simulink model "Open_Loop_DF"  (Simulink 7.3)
settings: Solver=ode3  StartTime=0.0  StopTime=500  FixedStep=0.002  RelTol=1e-3
undefined symbols (not defined in the file or in its folder): Acs, Av1, Bcs, Bv1, Ccs, Cv1, Dcs, Dv1

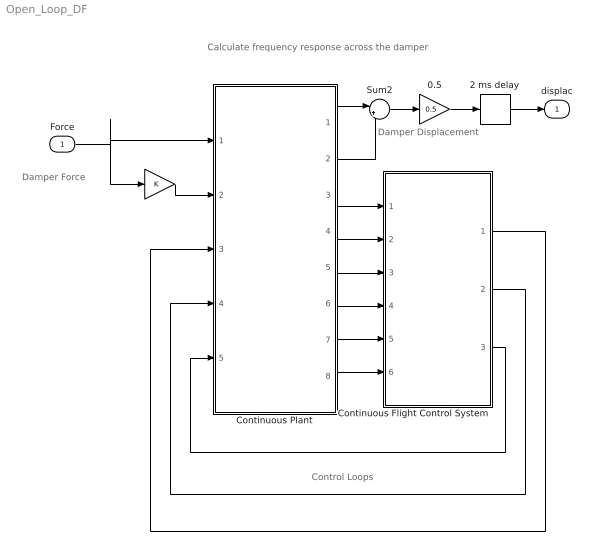
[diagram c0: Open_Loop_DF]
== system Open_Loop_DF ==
  note: Calculate frequency response across the damper
  note: Control Loops
  note: Damper Force
  note: Damper Displacement
  Force : Inport  OutDataType=sfix(16)  OutScaling=2^0
  "  " : Gain  ParameterDataType=sfix(16)  ParameterScaling=2^0  OutDataType=sfix(16)  OutScaling=2^0
  0.5 : Gain  Gain=0.5  ParameterDataType=sfix(16)  ParameterScaling=2^0  OutDataType=sfix(16)  OutScaling=2^0
  2 ms delay : TransportDelay  DelayTime=0.002  PadeOrder=2
  Continuous Flight Control System : Subsystem
  Continuous Plant : Subsystem
  Sum2 : Sum  Inputs=|++  OutDataType=sfix(16)  OutScaling=2^0
  displac : Outport  OutDataType=sfix(16)  OutScaling=2^0
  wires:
  Force/1 -> "  "/1, Continuous Plant/1(F-left)
  Sum2/1 -> 0.5/1
  0.5/1 -> 2 ms delay/1
  "  "/1 -> Continuous Plant/2(F-right)
  Continuous Plant/3(phi) -> Continuous Flight Control System/1(Phi)
  Continuous Plant/4(theta) -> Continuous Flight Control System/2(Theta)
  Continuous Plant/6(P) -> Continuous Flight Control System/4(P)
  Continuous Plant/7(Q) -> Continuous Flight Control System/5(Q)
  Continuous Plant/8(R) -> Continuous Flight Control System/6(R)
  Continuous Plant/5(psi) -> Continuous Flight Control System/3(Psi)
  Continuous Flight Control System/2(DQ-TVC) -> Continuous Plant/4(DQ)
  Continuous Flight Control System/3(DR-TVC) -> Continuous Plant/5(DR)
  Continuous Flight Control System/1(DP-TVC) -> Continuous Plant/3(DP)
  2 ms delay/1 -> displac/1
  Continuous Plant/1(dZ-Left) -> Sum2/1
  Continuous Plant/2(dZ-Rght) -> Sum2/2

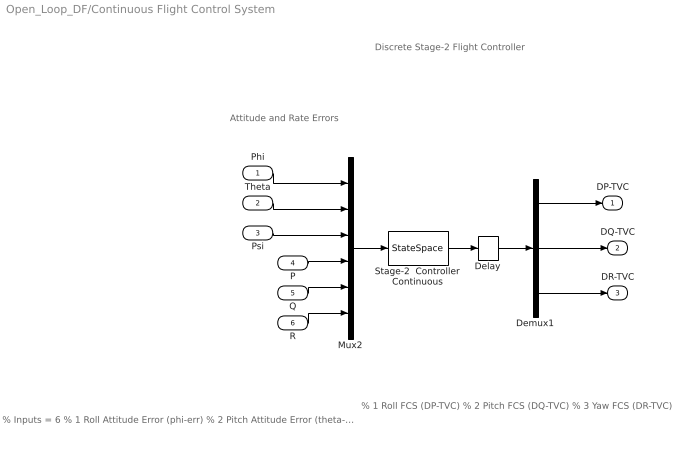
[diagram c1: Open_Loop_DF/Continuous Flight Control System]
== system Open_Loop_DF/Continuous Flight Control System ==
  note: % 1 Roll FCS (DP-TVC) % 2 Pitch FCS (DQ-TVC) % 3 Yaw FCS (DR-TVC)
  note: % Inputs = 6 % 1 Roll Attitude Error (phi-err) % 2 Pitch Attitude Error (theta-err) % 3 Yaw Attitude Error (psi-err) % 4 Roll Rate Error (p-err) % 5 Pitch Rate Error (q-err) % 6 Yaw Rate Error (r-err)
  note: Attitude and Rate Errors
  note: Discrete Stage-2 Flight Controller
  Phi : Inport  OutDataType=sfix(16)  OutScaling=2^0
  Theta : Inport  Port=2  OutDataType=sfix(16)  OutScaling=2^0
  Psi : Inport  Port=3  OutDataType=sfix(16)  OutScaling=2^0
  P : Inport  Port=4  OutDataType=sfix(16)  OutScaling=2^0
  Q : Inport  Port=5  OutDataType=sfix(16)  OutScaling=2^0
  R : Inport  Port=6  OutDataType=sfix(16)  OutScaling=2^0
  Delay : TransportDelay  DelayTime=0.04  PadeOrder=2
  Demux1 : Demux  Outputs=3
  Mux2 : Mux  Inputs=6
  Stage-2  Controller Continuous : StateSpace  A=Acs  B=Bcs  C=Ccs  D=Dcs
  DP-TVC : Outport  OutDataType=sfix(16)  OutScaling=2^0
  DQ-TVC : Outport  Port=2  OutDataType=sfix(16)  OutScaling=2^0
  DR-TVC : Outport  Port=3  OutDataType=sfix(16)  OutScaling=2^0
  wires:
  Demux1/3 -> DR-TVC/1
  Demux1/1 -> DP-TVC/1
  Demux1/2 -> DQ-TVC/1
  P/1 -> Mux2/4
  Stage-2  Controller Continuous/1 -> Delay/1
  Psi/1 -> Mux2/3
  Theta/1 -> Mux2/2
  Phi/1 -> Mux2/1
  R/1 -> Mux2/6
  Q/1 -> Mux2/5
  Mux2/1 -> Stage-2  Controller Continuous/1
  Delay/1 -> Demux1/1

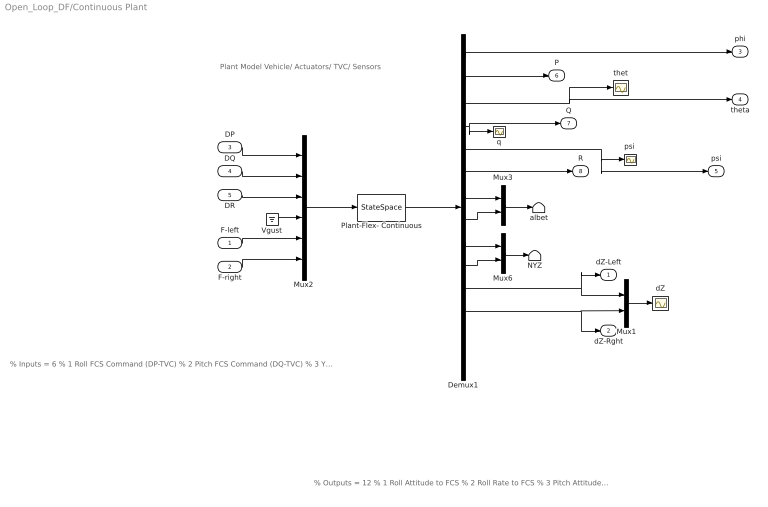
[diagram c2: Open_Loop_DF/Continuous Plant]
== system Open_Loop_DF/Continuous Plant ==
  note: % Outputs = 12 % 1 Roll Attitude to FCS % 2 Roll Rate to FCS % 3 Pitch Attitude to FCS % 4 Pitch Rate to FCS % 5 Yaw Attitude to FCS % 6 Yaw Rate to FCS % 7 Angle of Attack, alpha (rad) % 8 Angle of Sideslip, beta (rad) % 9 Normal Accelerometer, Nz (ft/sec^2) % 10 Lateral Accelerometer, Ny (ft/sec^2) % 11 Left Damper Extension (ft) % 12 Right Damper Extension (ft) % 13 Left Damper Rate (ft/sec) % 14 Right Damper Rate (ft/s)
  note: % Inputs = 6 % 1 Roll FCS Command (DP-TVC) % 2 Pitch FCS Command (DQ-TVC) % 3 Yaw FCS Command (DR-TVC) % 4 Wind-Gust Velocity (ft/sec) % 5 Left Coulomb Damper Force % 6 Right Coulomb Damper Force
  note: Plant Model Vehicle/ Actuators/ TVC/ Sensors
  F-left : Inport  OutDataType=sfix(16)  OutScaling=2^0
  F-right : Inport  Port=2  OutDataType=sfix(16)  OutScaling=2^0
  DP : Inport  Port=3  OutDataType=sfix(16)  OutScaling=2^0
  DQ : Inport  Port=4  OutDataType=sfix(16)  OutScaling=2^0
  DR : Inport  Port=5  OutDataType=sfix(16)  OutScaling=2^0
  Demux1 : Demux  Outputs=14
  Mux1 : Mux  Inputs=2
  Mux2 : Mux  Inputs=6
  Mux3 : Mux  Inputs=2
  Mux6 : Mux  Inputs=2
  NYZ : Terminator
  Plant-Flex- Continuous : StateSpace  A=Av1  B=Bv1  C=Cv1  D=Dv1
  Vgust : Ground
  albet : Terminator
  dZ : Scope
  "psi " : Scope
  q : Scope
  thet : Scope
  dZ-Left : Outport  OutDataType=sfix(16)  OutScaling=2^0
  dZ-Rght : Outport  Port=2  OutDataType=sfix(16)  OutScaling=2^0
  phi : Outport  Port=3  OutDataType=sfix(16)  OutScaling=2^0
  theta : Outport  Port=4  OutDataType=sfix(16)  OutScaling=2^0
  psi : Outport  Port=5  OutDataType=sfix(16)  OutScaling=2^0
  P : Outport  Port=6  OutDataType=sfix(16)  OutScaling=2^0
  Q : Outport  Port=7  OutDataType=sfix(16)  OutScaling=2^0
  R : Outport  Port=8  OutDataType=sfix(16)  OutScaling=2^0
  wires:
  Demux1/4 -> q/1, Q/1
  Demux1/5 -> "psi "/1, psi/1
  Demux1/1 -> phi/1
  Demux1/3 -> thet/1, theta/1
  Mux1/1 -> dZ/1
  Plant-Flex- Continuous/1 -> Demux1/1
  Demux1/10 -> Mux6/2
  Demux1/8 -> Mux3/2
  Demux1/6 -> R/1
  Demux1/2 -> P/1
  Vgust/1 -> Mux2/4
  Mux6/1 -> NYZ/1
  Mux3/1 -> albet/1
  Mux2/1 -> Plant-Flex- Continuous/1
  Demux1/12 -> Mux1/2, dZ-Rght/1
  Demux1/11 -> Mux1/1, dZ-Left/1
  Demux1/9 -> Mux6/1
  Demux1/7 -> Mux3/1
  DR/1 -> Mux2/3
  DQ/1 -> Mux2/2
  DP/1 -> Mux2/1
  F-right/1 -> Mux2/6
  F-left/1 -> Mux2/5
